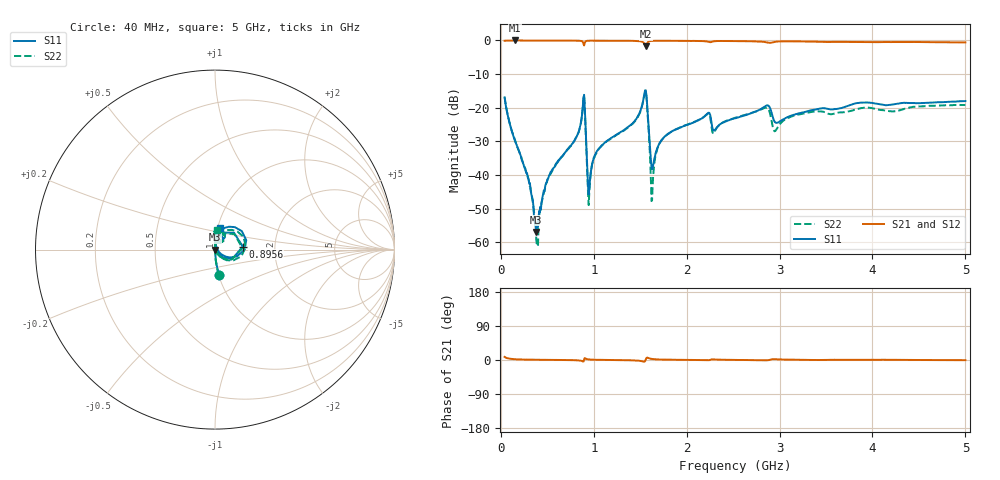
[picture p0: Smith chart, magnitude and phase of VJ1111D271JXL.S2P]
! VJ1111D271JXL
! DATE 02/15/2022  13:34
! CAPACITORS MOUNTED IN SERIES ON 25 MIL THICK MICROSTRIP SUBSTRATE
# GHz  S  MA  R  50.00
!  FREQ  S11M  S11A  S21M  S21A  S12M  S12A  S22M  S22A
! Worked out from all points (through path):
!   801 points, 40 MHz to 5 GHz, reference 50 ohm
!   highest |S21| = 0.00 dB at 151.6 MHz (marker M1); lowest = -1.7 dB at 1.559 GHz (marker M2)
!   lowest |S11| = -56.9 dB at 381 MHz (marker M3), VSWR 1.00, Z = 50.1 + j0.00362 ohm
!   |S11| at or under -10 dB: start of sweep to end of sweep
!   |S22| runs from -61.2 to -15.2 dB; largest |S21 - S12| = 0.011
!   S11 on the Smith chart (normalised r, x): 40 MHz: 1.01, -0.29; 895.6 MHz: 1.37, +0.05; 5 GHz: 1.03, +0.25
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0.04  0.1422 -80.6  0.9898 8.1  0.9897 8.3  0.1443 -81.0
0.1516  0.03229 -85.7  0.9996 2.1  0.9961 2.2  0.03317 -87.4
0.2942  0.008846 -81.1  0.9971 0.9  1 0.9  0.008995 -83.5
0.381  0.001425 1.4  0.9956 0.6  1.001 0.6  0.001093 -58.0
0.505  0.008728 79.6  0.9958 0.3  0.9992 0.4  0.00875 81.8
0.8026  0.03448 85.0  0.9924 -0.6  0.9974 -0.6  0.03475 83.8
0.8708  0.07324 74.6  0.9765 -2.5  0.9813 -2.6  0.07219 72.5
0.8956  0.1557 6.3  0.843 1.0  0.8479 0.9  0.1527 2.9
0.9328  0.01039 -40.1  0.9887 2.0  0.9942 1.9  0.009312 -49.2
0.9576  0.007964 64.5  0.9919 1.2  0.9981 1.2  0.007471 72.7
1.0506  0.02431 85.0  0.9944 0.4  0.9968 0.3  0.02394 85.4
1.559  0.182 16.5  0.8189 0.9  0.8228 0.8  0.1731 5.4
1.6272  0.01215 21.7  0.9858 2.7  0.99 2.6  0.004177 49.0
1.6954  0.02739 82.0  0.9891 1.4  0.9947 1.3  0.02716 90.7
2.2224  0.08198 76.5  0.9642 -0.7  0.9695 -0.9  0.08017 73.1
2.2968  0.04564 72.3  0.9731 1.5  0.9782 1.4  0.04314 77.0
2.52  0.06966 87.1  0.9783 0.2  0.984 0.0  0.07079 88.1
2.8548  0.1071 73.0  0.9418 -0.9  0.9464 -1.2  0.0999 67.2
2.954  0.06039 62.6  0.9553 2.1  0.9605 2.0  0.04523 72.7
3.3508  0.0923 85.2  0.9623 0.1  0.9676 -0.1  0.08704 88.6
4.1754  0.1098 77.4  0.9472 0.4  0.9546 0.2  0.08916 85.7
5  0.1255 76.7  0.9337 -0.4  0.9384 -0.6  0.1097 83.4
